| TEXAS INSTRUMENTS INCORPORATED
| Standard Linear and Logic Group
| IBIS Model of TXS01081BIT_IBIS
| 8-BIT BIDIRECTIONAL VOLTAGE-LEVEL TRANSLATOR WITH AUTO DIRECTION
| SENSING AND +/-15KV ESD PROTECTION
| This file contains package information for the following:
|  TSSOP 20-pin (PW) package as [Component] TXS01081BIT_IBIS_PW
|  QFN 20-pin (RGY) package as [Component] TXS01081BIT_IBIS_RGY
| This device can be powered at the following Vccs:
|  5 volt Vcc
|  3.3 volt Vcc
|  2.5 volt Vcc
|  1.8 volt Vcc
|  1.5 volt Vcc
|  1.2 volt Vcc
| This file provides unique models under the [Model Selector] for each Vcc.
| For operation at a specific Vcc, select the appropriate model after each
| [Model Selector] keyword.
[IBIS Ver]   3.2
[Comment char]  |_char
[File Name]   txs0108e.ibs
[File Rev]   1.0 | x_die
[Date]   May 9, 2009
[Source]   Data created from TI-SPICE simulations at TI-SLL.
[Notes]   The following is an IBIS list for the TXS0108E.
   Please contact sllibis@ti.com with questions and
   comments concerning SLL IBIS models.
   Pullup and Pulldown non-monotonic reflects circuit behavior
   IOB and IOA I/O buffers
[Disclaimer] Property of Texas Instruments Incorporated.  Unauthorized
   reproduction and/or distribution is strictly prohibited.
   This product is protected under copyright law.
   Created  2009, (C) Copyright  2009, Texas Instruments
   Incorporated, All Rights Reserved
   UNLESS THERE IS A SIGNED, WRITTEN AGREEMENT TO THE
   CONTRARY, TEXAS INSTRUMENTS (TI) IS PROVIDING THE IBIS
   MODELS  AND WITHOUT ANY WARRANTY, EXPRESSED OR
   IMPLIED.  TI assumes no liability for:
   1) the accuracy of the IBIS models provided to your
   company;
   2) the proper functioning of these IBIS Models in your
   design or for any resulting applications; or
   3) infringement of patents, copyrights or intellectual
   property rights resulting from your use of these IBIS
   models.
   TI provides IBIS Models as a service to our customers.
   You and your company shall not distribute, sell or give
   these models to anyone else without prior written
   permission from TI.
   TI reserves the right to make changes to our products or
   to discontinue any semiconductor product or service
   without notice, and advises our customers to obtain the
   latest version of relevant information to verify, before
   placing orders, that the information being relied on is
   current.
   Please be aware that your receipt and use of the IBIS
   information provided shall serve as acceptance of these
   terms and conditions.  If you do not accept these terms,
   you should return or destroy the IBIS models and any
   other accompanying information immediately.
| Component TXS0108E_PW 20-PIN TSSOP
[Component]   TXS0108E_PW
[Manufacturer]   Texas Instruments, Inc.
[Package]
|   typ   min   max
R_pkg   5.000e-02   4.200e-02   6.000e-02
L_pkg   2.802e-09   2.248e-09   3.553e-09
C_pkg   3.170e-13   2.020e-13   4.430e-13
[Pin]   signal_name   model_name   R_pin   L_pin   C_pin
1   A1   TXS0108_IOA   5.500e-02   3.461e-09   4.400e-13
2   VCCA   POWER   5.500e-02   3.150e-09   4.010e-13
3   A2   TXS0108_IOA   4.200e-02   2.619e-09   3.020e-13
4   A3   TXS0108_IOA   4.500e-02   2.273e-09   2.020e-13
5   A4   TXS0108_IOA   4.500e-02   2.248e-09   2.240e-13
6   A5   TXS0108_IOA   4.500e-02   2.273e-09   2.260e-13
7   A6   TXS0108_IOA   4.400e-02   2.323e-09   2.050e-13
8   A7   TXS0108_IOA   4.600e-02   2.704e-09   3.070e-13
9   A8   TXS0108_IOA   6.000e-02   3.265e-09   4.110e-13
10   OE   TXS0108_IN   5.700e-02   3.506e-09   4.360e-13
11   GND   GND   5.800e-02   3.553e-09   4.370e-13
12   B8   TXS0108_IOB   5.800e-02   3.193e-09   4.050e-13
13   B7   TXS0108_IOB   4.200e-02   2.704e-09   3.110e-13
14   B6   TXS0108_IOB   4.600e-02   2.392e-09   2.100e-13
15   B5   TXS0108_IOB   4.700e-02   2.334e-09   2.290e-13
16   B4   TXS0108_IOB   4.700e-02   2.300e-09   2.270e-13
17   B3   TXS0108_IOB   4.700e-02   2.349e-09   2.070e-13
18   B2   TXS0108_IOB   4.500e-02   2.677e-09   3.060e-13
19   VCCB   POWER   6.000e-02   3.235e-09   4.060e-13
20   B1   TXS0108_IOB   5.600e-02   3.487e-09   4.430e-13
| Component TXS0108E_RGY 20-PIN QFN
[Component]   TXS0108E_RGY
[Manufacturer]   Texas Instruments, Inc.
[Package]
|   typ   min   max
R_pkg   5.000e-02   4.600e-02   5.500e-02
L_pkg   1.119e-09   1.025e-09   1.227e-09
C_pkg   3.520e-13   3.440e-13   3.630e-13
[Pin]   signal_name   model_name   R_pin   L_pin   C_pin
1   A1   TXS0108_IOA   5.200e-02   1.167e-09   3.600e-13
2   VCCA   POWER   4.700e-02   1.049e-09   3.440e-13
3   A2   TXS0108_IOA   4.700e-02   1.055e-09   3.450e-13
4   A3   TXS0108_IOA   5.000e-02   1.119e-09   3.500e-13
5   A4   TXS0108_IOA   5.500e-02   1.227e-09   3.600e-13
6   A5   TXS0108_IOA   5.200e-02   1.167e-09   3.550e-13
7   A6   TXS0108_IOA   4.900e-02   1.087e-09   3.480e-13
8   A7   TXS0108_IOA   4.700e-02   1.054e-09   3.460e-13
9   A8   TXS0108_IOA   4.900e-02   1.091e-09   3.490e-13
10   OE   TXS0108_IN   5.300e-02   1.184e-09   3.620e-13
11   GND   GND   5.300e-02   1.181e-09   3.600e-13
12   B8   TXS0108_IOB   5.000e-02   1.108e-09   3.490e-13
13   B7   TXS0108_IOB   4.800e-02   1.075e-09   3.470e-13
14   B6   TXS0108_IOB   5.000e-02   1.107e-09   3.490e-13
15   B5   TXS0108_IOB   5.400e-02   1.200e-09   3.620e-13
16   B4   TXS0108_IOB   5.100e-02   1.141e-09   3.570e-13
17   B3   TXS0108_IOB   4.700e-02   1.043e-09   3.440e-13
18   B2   TXS0108_IOB   4.600e-02   1.025e-09   3.440e-13
19   VCCB   POWER   4.900e-02   1.090e-09   3.490e-13
20   B1   TXS0108_IOB   5.400e-02   1.204e-09   3.630e-13
| Component TXS0108E_ZXY 20-PIN u*Jr BGA
[Component]   TXS0108E_ZXY
[Manufacturer]   Texas Instruments, Inc.
[Package]
|   typ   min   max
R_pkg   0.057703   0.05127   0.06781
L_pkg   1.1577665n  0.99154n   1.48216n
C_pkg   0.1802725p  0.13673p   0.22855p
[Pin]   signal_name   model_name   R_pin   L_pin   C_pin
1   A8   TXS0108_IOA   0.05373   1.01871n   0.15665p
2   A7   TXS0108_IOA   0.06276   1.39916n   0.21753p
3   A6   TXS0108_IOA   0.05433   1.01804n   0.18684p
4   A5   TXS0108_IOA   0.06043   1.35595n   0.22385p
5   A4   TXS0108_IOA   0.05268   0.99154n   0.18368p
6   A3   TXS0108_IOA   0.05974   1.35105n   0.21539p
7   A2   TXS0108_IOA   0.05308   1.00780n   0.16664p
8   VCCA   POWER   0.05705   1.02274n   0.16511p
9   A1   TXS0108_IOA   0.05192   1.03338n   0.13766p
10   B1   TXS0108_IOB   0.05127   1.02319n   0.13673p
11   VCCB   POWER   0.06180   1.16248n   0.14894p
12   B2   TXS0108_IOB   0.05734   1.07561n   0.17217p
13   B3   TXS0108_IOB   0.06444   1.42639n   0.22198p
14   B4   TXS0108_IOB   0.05770   1.07442n   0.18915p
15   B5   TXS0108_IOB   0.06564   1.44558n   0.22855p
16   B6   TXS0108_IOB   0.05938   1.10463n   0.19337p
17   B7   TXS0108_IOB   0.06781   1.48216n   0.22458p
18   B8   TXS0108_IOB   0.05895   1.10793n   0.16240p
19   GND   GND   0.05168   1.02154n   0.13715p
20   OE   TXS0108_IN   0.05233   1.03303n   0.13708p
| Component TXS0108E_NME 20-PIN u*Jr BGA
[Component]   TXS0108E_NME
[Manufacturer]   Texas Instruments, Inc.
[Package]
|   typ   min   max
R_pkg   0.057703   0.05127   0.06781
L_pkg   1.1577665n  0.99154n   1.48216n
C_pkg   0.1802725p  0.13673p   0.22855p
[Pin]   signal_name   model_name   R_pin   L_pin   C_pin
1   A8   TXS0108_IOA   0.05373   1.01871n   0.15665p
2   A7   TXS0108_IOA   0.06276   1.39916n   0.21753p
3   A6   TXS0108_IOA   0.05433   1.01804n   0.18684p
4   A5   TXS0108_IOA   0.06043   1.35595n   0.22385p
5   A4   TXS0108_IOA   0.05268   0.99154n   0.18368p
6   A3   TXS0108_IOA   0.05974   1.35105n   0.21539p
7   A2   TXS0108_IOA   0.05308   1.00780n   0.16664p
8   VCCA   POWER   0.05705   1.02274n   0.16511p
9   A1   TXS0108_IOA   0.05192   1.03338n   0.13766p
10   B1   TXS0108_IOB   0.05127   1.02319n   0.13673p
11   VCCB   POWER   0.06180   1.16248n   0.14894p
12   B2   TXS0108_IOB   0.05734   1.07561n   0.17217p
13   B3   TXS0108_IOB   0.06444   1.42639n   0.22198p
14   B4   TXS0108_IOB   0.05770   1.07442n   0.18915p
15   B5   TXS0108_IOB   0.06564   1.44558n   0.22855p
16   B6   TXS0108_IOB   0.05938   1.10463n   0.19337p
17   B7   TXS0108_IOB   0.06781   1.48216n   0.22458p
18   B8   TXS0108_IOB   0.05895   1.10793n   0.16240p
19   GND   GND   0.05168   1.02154n   0.13715p
20   OE   TXS0108_IN   0.05233   1.03303n   0.13708p
| Model TXS0108_IN
[Model Selector]   TXS0108_IN
TXS0108_IN_50   5 volt Vcc
TXS0108_IN_33   3.3 volt Vcc
TXS0108_IN_25   2.5 volt Vcc
TXS0108_IN_18   1.8 volt Vcc
TXS0108_IN_15A   1.5 volt Vcc
TXS0108_IN_12A   1.2 volt Vcc
| Model TXS0108_IOB
[Model Selector]   TXS0108_IOB
TXS0108_IOB_OS_50   5 volt Vcc
TXS0108_IOB_OS_33   3.3 volt Vcc
TXS0108_IOB_OS_25   2.5 volt Vcc
TXS0108_IOB_OS_18   1.8 volt Vcc
TXS0108_IOB_OS_15A   1.5 volt Vcc
TXS0108_IOB_OS_12A   1.2 volt Vcc
| Model TXS0108_IOA
[Model Selector]   TXS0108_IOA
TXS0108_IOA_OS_50   5 volt Vcc
TXS0108_IOA_OS_33   3.3 volt Vcc
TXS0108_IOA_OS_25   2.5 volt Vcc
TXS0108_IOA_OS_18   1.8 volt Vcc
TXS0108_IOA_OS_15A   1.5 volt Vcc
TXS0108_IOA_OS_12A   1.2 volt Vcc
| Models and submodels in the file (18): TXS0108_IN_50 (Input), TXS0108_IN_33 (Input), TXS0108_IN_25 (Input), TXS0108_IN_18 (Input), TXS0108_IN_15A (Input), TXS0108_IN_12A (Input), TXS0108_IOB_OS_50 (I/O), TXS0108_IOB_OS_33 (I/O), TXS0108_IOB_OS_25 (I/O), TXS0108_IOB_OS_18 (I/O), TXS0108_IOB_OS_15A (I/O), TXS0108_IOB_OS_12A (I/O), TXS0108_IOA_OS_50 (I/O), TXS0108_IOA_OS_33 (I/O), TXS0108_IOA_OS_25 (I/O), TXS0108_IOA_OS_18 (I/O), TXS0108_IOA_OS_15A (I/O), TXS0108_IOA_OS_12A (I/O)
